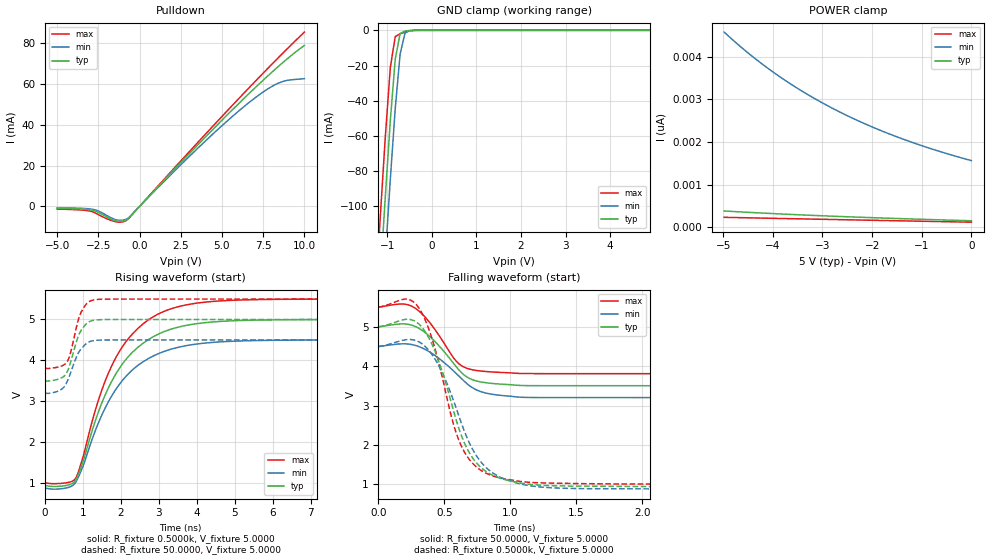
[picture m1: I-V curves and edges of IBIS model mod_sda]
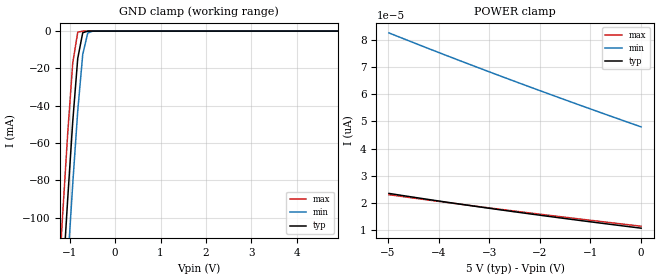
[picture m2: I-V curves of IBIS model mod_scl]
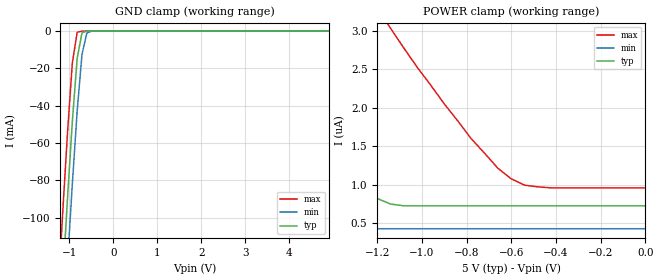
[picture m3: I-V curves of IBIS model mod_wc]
| IBIS (I/O, Buffer, Information, Specification) Model, officially
| electronic behavioral standard for Buffer structures of digital pins.
[IBIS ver]  4.0
[File name] m24c08_fb3_tssop8.ibs
[File Rev]  1.0
[Date]   23 Oct 2014
[Source]   CAD & Design Services (Catania) - STMicroelectronics
[Notes]
   (Note1)  This IBIS model includes the TSSOP8 package data
   (Note2)  This IBIS model has some Notes about the non-monotonicity
   of the I-V curves, but they are not indicative of problems
   inside the model;
[Copyright] (c) 2014 STMicroelectronics
|   Component M24C08
[Component] M24C08
[Manufacturer] STMicroelectronics
[Package]
| variable   typ   min   max
R_pkg   0.0   0.0   0.0
L_pkg   0.0H   0.0H   0.0H
C_pkg   0.0F   0.0F   0.0F
[Pin]  signal_name   model_name   R_pin   L_pin   C_pin
1   1NC   NC   NA   NA   NA
2   2NC   NC   NA   NA   NA
3   3NC   NC   NA   NA   NA
4   VSS   GND   NA   NA   NA
5   SDA   mod_sda   NA   NA   NA
6   SCL   mod_scl   NA   NA   NA
7   WCN   mod_wc   NA   NA   NA
8   VCC   POWER   NA   NA   NA
[Package Model]  182696_TSSOP8
[Define Package Model]  182696_TSSOP8
[Manufacturer]  STMicroelectronics
[OEM]  STMicroelectronics
[Description]  8 pin TSSOP package
[Number Of Pins]  8
[Pin Numbers]
|Pin Num   Terminal Name
1   | net1
2   | net2
3   | net3
4   | net4_GND
5   | net5
6   | net6
7   | net7
8   | net8_VDD
[Model Data]
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[End Model Data]
[End Package Model]
| Models and submodels in the file (3): mod_sda (I/O_open_drain), mod_scl (Input), mod_wc (Input)
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|   Model mod_sda
[Model]   mod_sda
Model_type I/O_open_drain
Polarity   Non-Inverting
Vinl   =   1.500V
Vinh   =   3.500V
Vmeas  =   2.500V
Cref   =   10pF
Rref   =   1k
Vref   =   5.000V
C_comp   2.024pF   1.846pF   2.119pF
[Temperature Range]  25.0000   85.0000   -40.0000
[Voltage Range]   5.0000V   4.5000V   5.5000V
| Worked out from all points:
|   slope of the pulldown table from 0 to 0.75 V, typ, clamps not added: 115 ohm
|   GND clamp passes 1 mA (typ) near -0.65 V on its own axis
|   rising waveform, R_fixture 0.5000k, V_fixture 5.0000: 20-80 % time 1.22ns typ, 1.24ns min, 1.18ns max; typ from 0.938 V to 5 V
|   rising waveform, R_fixture 50.0000, V_fixture 5.0000: 20-80 % time 310ps typ, 344ps min, 282ps max; typ from 3.5 V to 5 V
|   falling waveform, R_fixture 50.0000, V_fixture 5.0000: 20-80 % time 234ps typ, 267ps min, 209ps max; typ from 5 V to 3.5 V
|   falling waveform, R_fixture 0.5000k, V_fixture 5.0000: 20-80 % time 247ps typ, 277ps min, 223ps max; typ from 5 V to 0.938 V
[Pulldown]
|Voltage   I(typ)   I(min)   I(max)
-5V       -929uA     -780uA     -1.317mA
-2.92V    -1.818mA   -1.343mA   -2.458mA
-2.44V    -3.202mA   -2.474mA   -4.275mA
-1.48V    -6.968mA   -6.444mA   -7.468mA
-840mV    -6.801mA   -6.376mA   -7.121mA
-680mV    -5.837mA   -5.734mA   -6.086mA
3.96V     33.76mA    31.85mA    35.14mA
6.68V     55.71mA    51.26mA    58.56mA
7.64V     63.03mA    56.95mA    66.61mA
8.44V     68.86mA    60.59mA    73.19mA
9.08V     73.27mA    62.04mA    78.36mA
10V       79.03mA    62.7mA     85.6mA
[GND_clamp]
|Voltage   I(typ)   I(min)   I(max)
-5V       -1.852A    -1.883A    -1.821A
-1.26V    -184.5mA   -219.6mA   -150.1mA
-1.15V    -138.3mA   -173.3mA   -103.9mA
-1.04V    -93.46mA   -128.1mA   -59.71mA
-930mV    -51.3mA    -84.56mA   -21.15mA
-820mV    -16.44mA   -44.56mA   -3.581mA
-710mV    -1.796mA   -13.44mA   -1.965mA
-600mV    -344.1uA   -1.474mA   -1.014mA
-490mV    -86.89uA   -222.4uA   -233.3uA
-270mV    -216.5nA   -2.636uA   -23.44nA
4.9V      151.8pA    1.696nA    108.3pA
[POWER_clamp]
|Voltage   I(typ)   I(min)   I(max)
-4.98V    384.3pA    4.576nA    235.8pA
-4.5V     353pA      4.089nA    224.3pA
-3.96V    321.1pA    3.612nA    211.6pA
-3.42V    292.3pA    3.199nA    199.1pA
-2.82V    263.2pA    2.804nA    185.3pA
-2.16V    234.3pA    2.435nA    170.2pA
-1.5V     207.9pA    2.121nA    155.3pA
-780mV    181.5pA    1.831nA    139.1pA
0V        155.1pA    1.564nA    121.6pA
[Ramp]
| variable   typ   min   max
dV/dt_r   0.8984/0.3688n   0.7792/0.4143n   1.0146/0.3276n
dV/dt_f   0.8780/0.2890n   0.7792/0.3019n   1.0146/0.2328n
R_load = 50.0000
[Rising Waveform]
R_fixture= 0.5000k
V_fixture= 5.0000
V_fixture_min= 4.5000
V_fixture_max= 5.5000
|time   V(typ)   V(min)   V(max)
0s        937.7mV    875.3mV    1.004V
540ps     934.5mV    872.8mV    999.8mV
820ps     1.077V     1.026V     1.128V
1ns       1.5V       1.393V     1.611V
1.42ns    2.758V     2.487V     3.048V
1.82ns    3.585V     3.217V     3.975V
2.32ns    4.209V     3.777V     4.658V
3.02ns    4.656V     4.175V     5.149V
4.7ns     4.957V     4.457V     5.459V
10ns      5V         4.5V       5.5V
[Rising Waveform]
R_fixture= 50.0000
V_fixture= 5.0000
V_fixture_min= 4.5000
V_fixture_max= 5.5000
|time   V(typ)   V(min)   V(max)
0s        3.503V     3.201V     3.809V
370ps     3.544V     3.256V     3.841V
490ps     3.6V       3.331V     3.883V
570ps     3.684V     3.445V     3.942V
670ps     3.923V     3.672V     4.159V
870ps     4.56V      4.156V     4.949V
950ps     4.723V     4.275V     5.165V
1.11ns    4.909V     4.422V     5.395V
1.31ns    4.984V     4.486V     5.482V
10ns      5V         4.5V       5.5V
[Falling Waveform]
R_fixture= 50.0000
V_fixture= 5.0000
V_fixture_min= 4.5000
V_fixture_max= 5.5000
|time   V(typ)   V(min)   V(max)
0s        5V         4.5V       5.5V
190ps     5.074V     4.567V     5.579V
290ps     4.992V     4.518V     5.448V
430ps     4.624V     4.27V      4.926V
570ps     4.072V     3.878V     4.21V
650ps     3.775V     3.62V      3.975V
710ps     3.66V      3.459V     3.91V
790ps     3.591V     3.339V     3.872V
1.05ns    3.514V     3.218V     3.818V
10ns      3.503V     3.201V     3.809V
[Falling Waveform]
R_fixture= 0.5000k
V_fixture= 5.0000
V_fixture_min= 4.5000
V_fixture_max= 5.5000
|time   V(typ)   V(min)   V(max)
0s        5V         4.5V       5.5V
200ps     5.185V     4.667V     5.703V
290ps     5.118V     4.645V     5.557V
350ps     4.903V     4.517V     5.218V
430ps     4.376V     4.177V     4.442V
570ps     2.866V     3.126V     2.518V
650ps     2.065V     2.367V     1.832V
810ps     1.34V      1.446V     1.292V
1.07ns    1.035V     1.013V     1.074V
10ns      937.7mV    875.3mV    1.004V
|   Model mod_scl
[Model]   mod_scl
Model_type Input
Vinl   =   1.500V
Vinh   =   3.500V
C_comp   1.762pF   1.683pF   1.932pF
[Temperature Range]  25.0000   85.0000   -40.0000
[Voltage Range]   5.0000V   4.5000V   5.5000V
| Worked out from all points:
|   GND clamp passes 1 mA (typ) near -0.71 V on its own axis
[GND_clamp]
|Voltage   I(typ)   I(min)   I(max)
-5V       -1.81A     -1.842A    -1.778A
-1.26V    -178.8mA   -214.1mA   -143mA
-1.15V    -133.6mA   -168.8mA   -97.85mA
-1.04V    -89.77mA   -124.5mA   -54.7mA
-930mV    -48.59mA   -81.99mA   -17.17mA
-820mV    -14.68mA   -42.87mA   -624.4uA
-710mV    -882.5uA   -12.5mA    -4.426uA
-600mV    -18.77uA   -1.029mA   -29.45nA
-490mV    -372.8nA   -42.06uA   -196.9pA
4.9V      10.41pA    50.62pA    10.07pA
[POWER_clamp]
|Voltage   I(typ)   I(min)   I(max)
-4.98V    23.46pA    82.67pA    22.99pA
-3.78V    20.06pA    73.87pA    19.98pA
-2.58V    16.89pA    65.38pA    17.13pA
-1.38V    13.9pA     57.16pA    14.39pA
0V        10.64pA    47.99pA    11.36pA
|   Model mod_wc
[Model]   mod_wc
Model_type Input
Vinl   =   1.500V
Vinh   =   3.500V
C_comp   1.762pF   1.683pF   1.932pF
[Temperature Range]  25.0000   85.0000   -40.0000
[Voltage Range]   5.0000V   4.5000V   5.5000V
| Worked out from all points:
|   GND clamp passes 1 mA (typ) near -0.71 V on its own axis
[GND_clamp]
|Voltage   I(typ)   I(min)   I(max)
-5V       -1.81A     -1.842A    -1.778A
-1.26V    -178.8mA   -214.1mA   -143mA
-1.15V    -133.6mA   -168.8mA   -97.85mA
-1.04V    -89.77mA   -124.5mA   -54.7mA
-930mV    -48.59mA   -81.99mA   -17.17mA
-820mV    -14.68mA   -42.87mA   -624.4uA
-710mV    -882.5uA   -12.5mA    -4.426uA
-600mV    -18.77uA   -1.029mA   -29.45nA
-490mV    -372.8nA   -42.06uA   -196.9pA
4.9V      10.41pA    50.62pA    10.07pA
[POWER_clamp]
|Voltage   I(typ)   I(min)   I(max)
-4.98V    12.45uA    7.203uA    21.47uA
-3.3V     6.708uA    3.037uA    13.54uA
-2.88V    5.017uA    2.187uA    11.06uA
-2.28V    3.354uA    1.92uA     7.431uA
-1.98V    2.96uA     1.451uA    5.864uA
-1.5V     1.758uA    535nA      4.302uA
-1.26V    987.6nA    430.2nA    3.531uA
-1.14V    750.1nA    430.2nA    3.031uA
-780mV    727.1nA    430.2nA    1.6uA
-600mV    727.1nA    430.2nA    1.077uA
-420mV    727.1nA    430.2nA    959.9nA
0V        727.1nA    430.2nA    959.9nA
